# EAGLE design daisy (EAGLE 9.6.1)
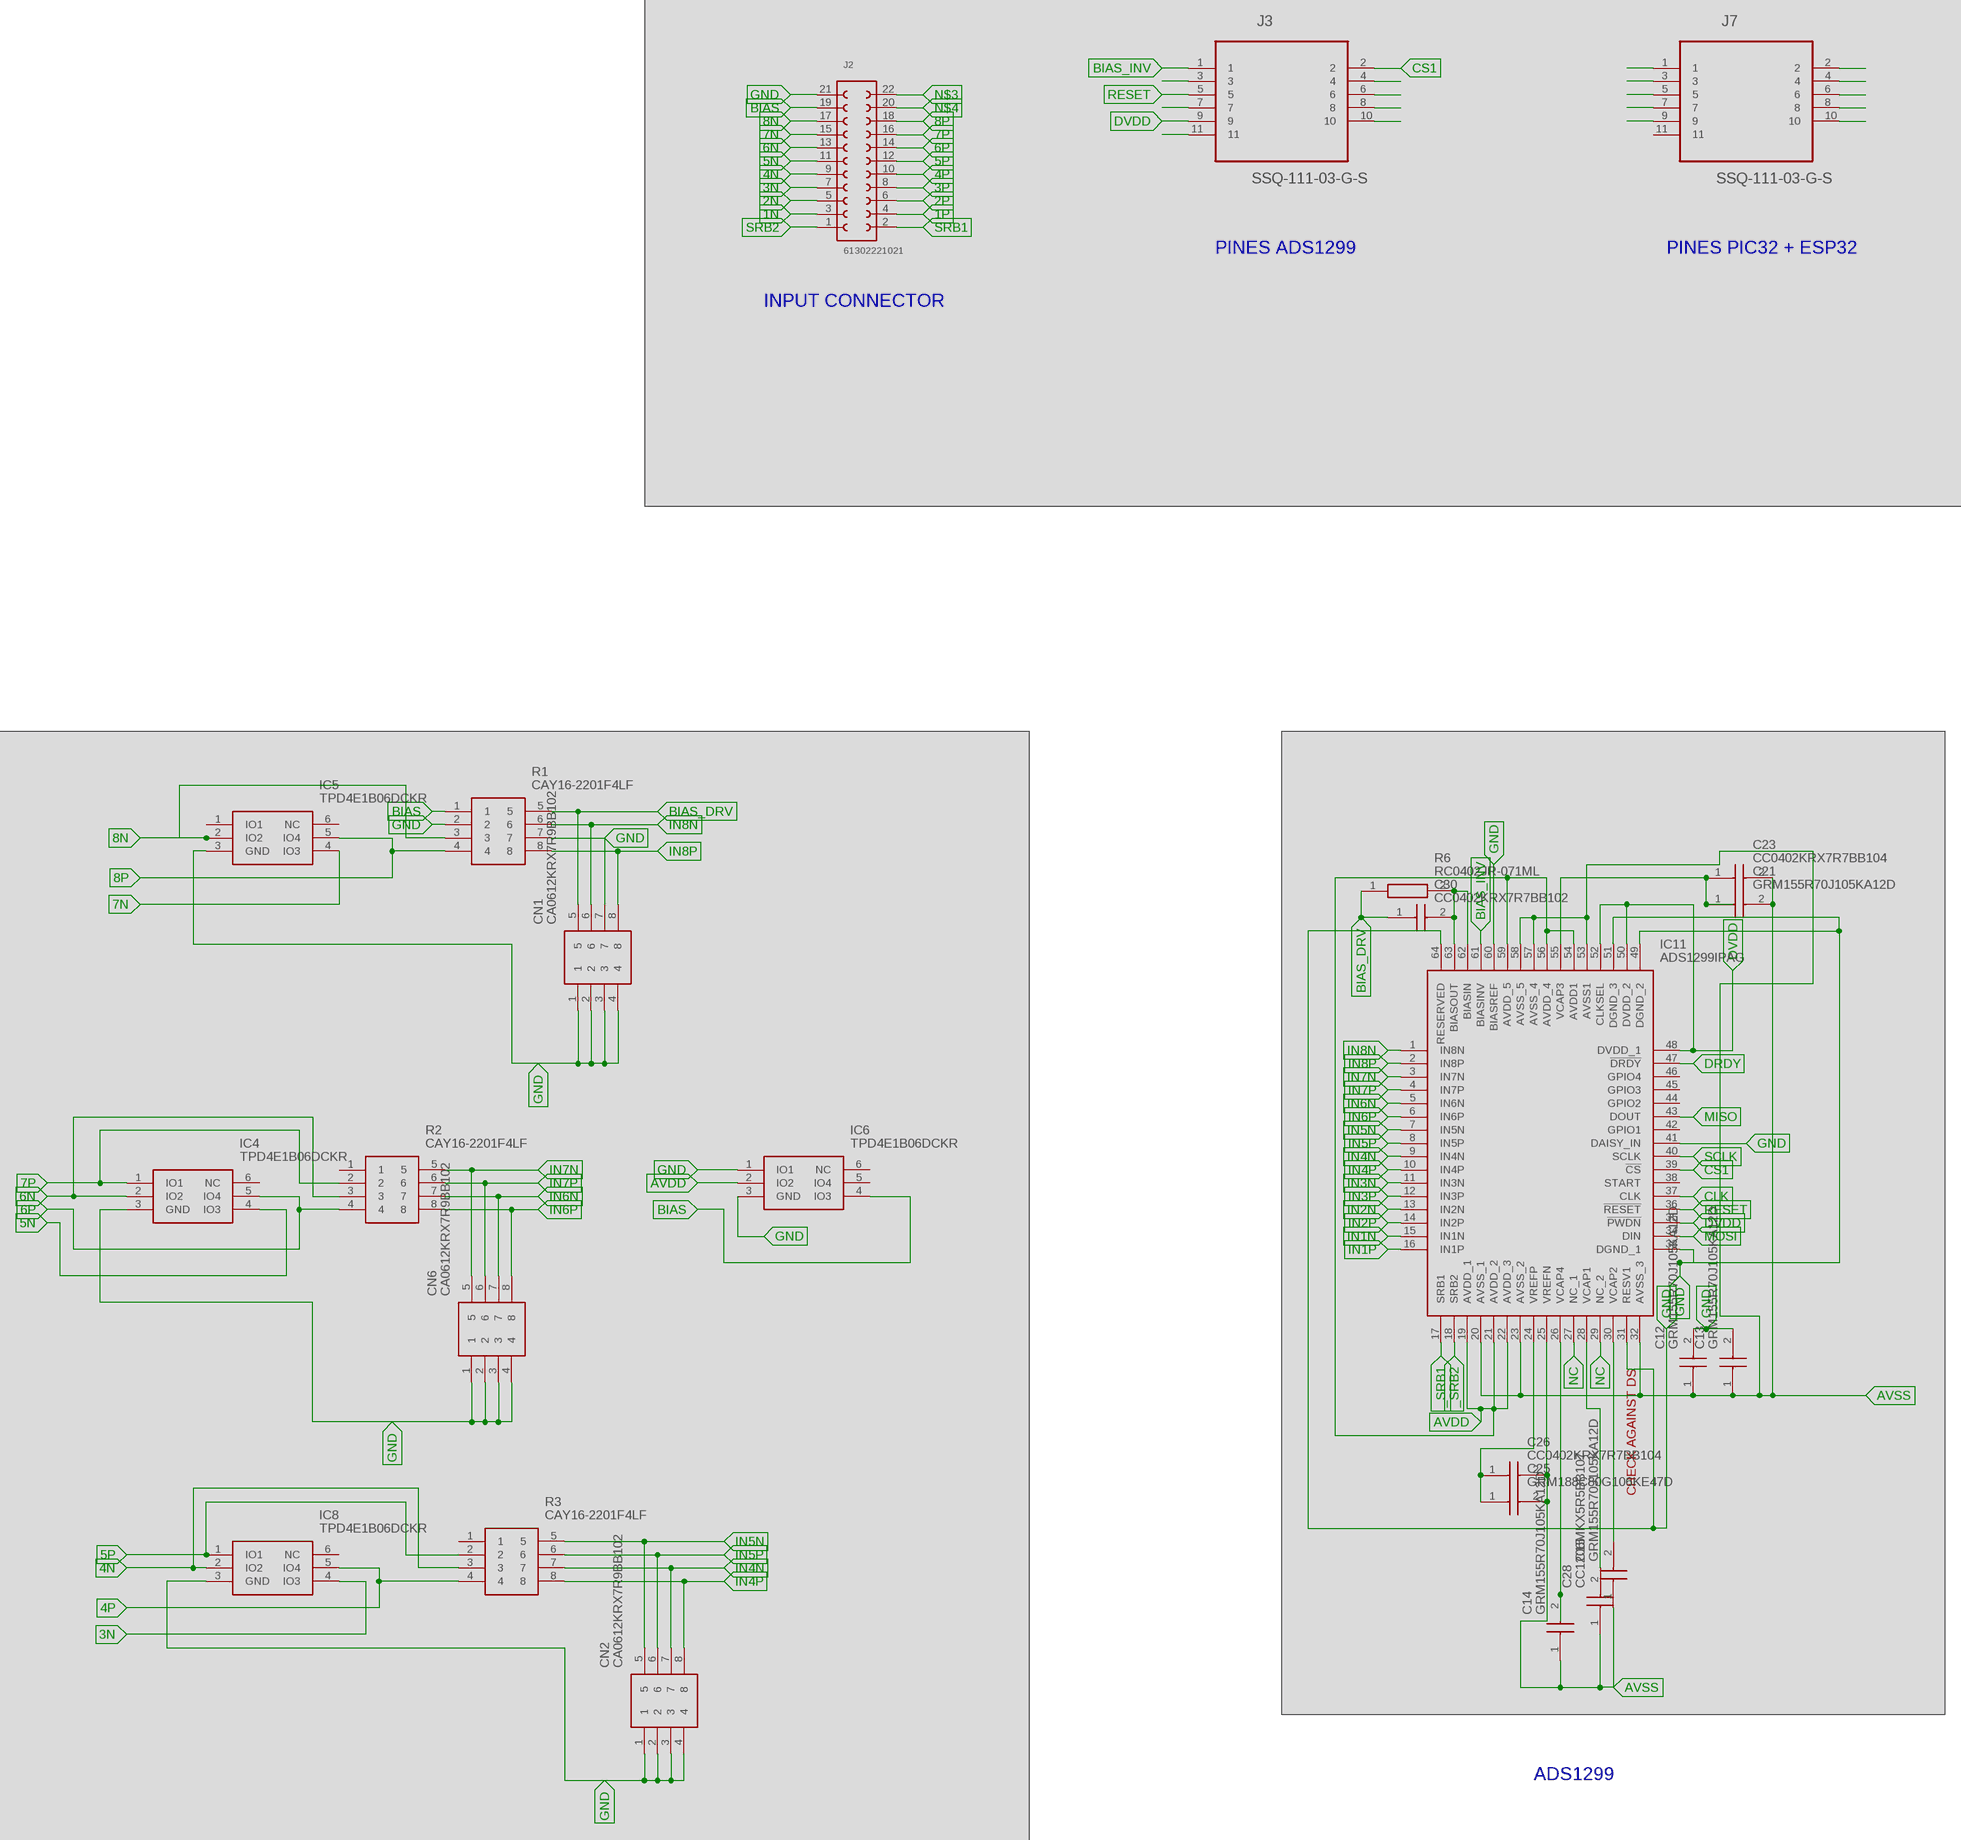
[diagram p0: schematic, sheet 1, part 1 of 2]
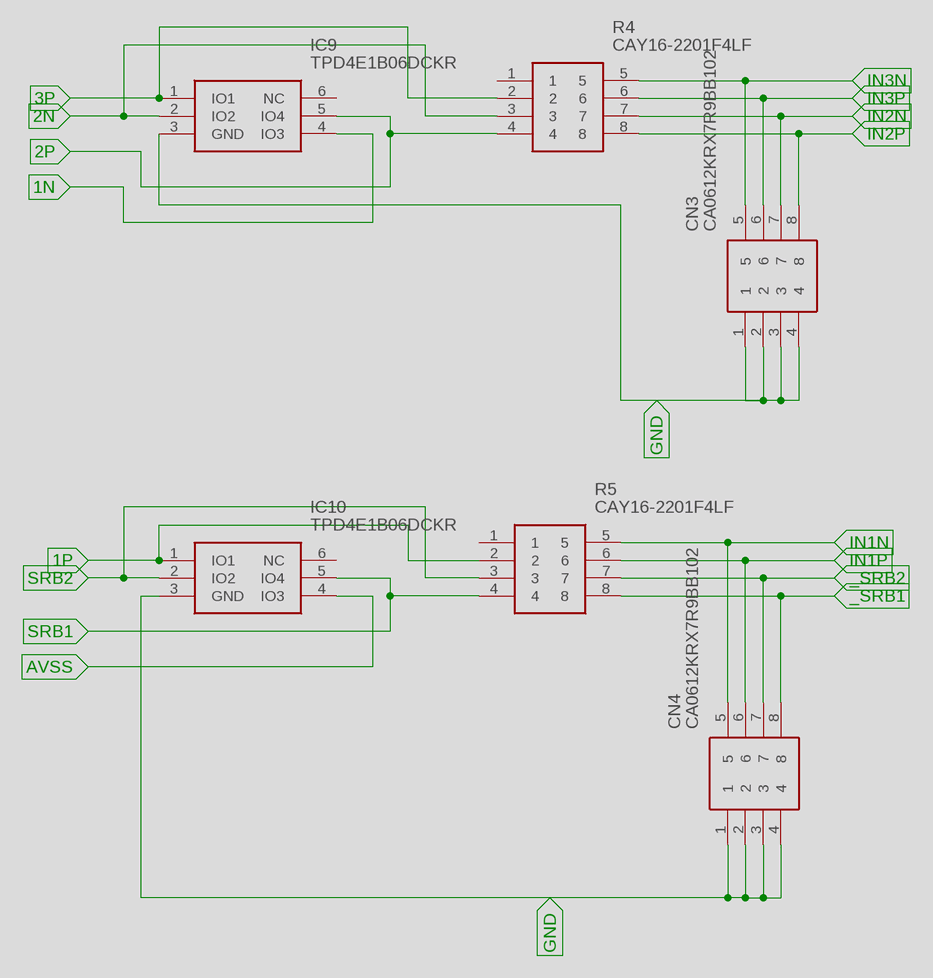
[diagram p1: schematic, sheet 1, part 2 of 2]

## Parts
C12  GRM155R70J105KA12D  [CAPC1005X55N]
C13  GRM155R70J105KA12D  [CAPC1005X55N]
C14  GRM155R70J105KA12D  [CAPC1005X55N]
C15  GRM155R70J105KA12D  [CAPC1005X55N]
C21  GRM155R70J105KA12D  [CAPC1005X55N]
C23  CC0402KRX7R7BB104  [CAPC1005X55N]
C25  GRM188C80G106KE47D  [CAPC1608X90N]
C26  CC0402KRX7R7BB104  [CAPC1005X55N]
C28  CC1206MKX5R5BB107  [CAPC3216X125N]
C30  CC0402KRX7R7BB102  [CAPC1005X55N]
CN1  CA0612KRX7R9BB102  [CA0612KRX7R9BB102]
CN2  CA0612KRX7R9BB102  [CA0612KRX7R9BB102]
CN3  CA0612KRX7R9BB102  [CA0612KRX7R9BB102]
CN4  CA0612KRX7R9BB102  [CA0612KRX7R9BB102]
CN6  CA0612KRX7R9BB102  [CA0612KRX7R9BB102]
IC4  TPD4E1B06DCKR  [SOT65P210X110-6N]
IC5  TPD4E1B06DCKR  [SOT65P210X110-6N]
IC6  TPD4E1B06DCKR  [SOT65P210X110-6N]
IC8  TPD4E1B06DCKR  [SOT65P210X110-6N]
IC9  TPD4E1B06DCKR  [SOT65P210X110-6N]
IC10  TPD4E1B06DCKR  [SOT65P210X110-6N]
IC11  ADS1299IPAG  [QFP50P1200X1200X120-64N]
J2  61302221021  [61302221021]
J3  SSQ-111-03-G-S  [SAMTEC_SSQ-111-03-G-S]
J7  SSQ-111-03-G-S  [SAMTEC_SSQ-111-03-G-S]
R1  CAY16-2201F4LF  [RESCAX80P160X320X60-8N]
R2  CAY16-2201F4LF  [RESCAX80P160X320X60-8N]
R3  CAY16-2201F4LF  [RESCAX80P160X320X60-8N]
R4  CAY16-2201F4LF  [RESCAX80P160X320X60-8N]
R5  CAY16-2201F4LF  [RESCAX80P160X320X60-8N]
R6  RC0402JR-071ML  [RESC1005X40N]

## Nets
1N: IC9.4(IO3) J2.3
1P: IC10.1(IO1) J2.4 R5.2
2N: IC9.2(IO2) J2.5 R4.3
2P: IC9.5(IO4) J2.6 R4.4
3N: IC8.4(IO3) J2.7
3P: IC9.1(IO1) J2.8 R4.2
3V3_ESP: J7.2
4N: IC8.2(IO2) J2.9 R3.3
4P: IC8.5(IO4) J2.10 R3.4
5N: IC4.4(IO3) J2.11
5P: IC8.1(IO1) J2.12 R3.2
6N: IC4.2(IO2) J2.13 R2.3
6P: IC4.5(IO4) J2.14 R2.4
7N: IC5.4(IO3) J2.15
7P: IC4.1(IO1) J2.16 R2.2
8N: IC5.2(IO2) J2.17 R1.3
8P: IC5.5(IO4) J2.18 R1.4
_SRB1: CN4.8 IC11.17(SRB1) R5.8
_SRB2: CN4.7 IC11.18(SRB2) R5.7
AVDD: IC6.2(IO2) IC11.19(AVDD_1) IC11.21(AVDD_2) IC11.22(AVDD_3) IC11.54(AVDD1) IC11.56(AVDD_4) IC11.59(AVDD_5) J3.10
AVSS: C12.1 C13.1 C14.1 C15.1 C21.2 C23.2 C25.2 C26.2 C28.1 IC10.4(IO3) IC11.20(AVSS_1) IC11.23(AVSS_2) IC11.25(VREFN) IC11.32(AVSS_3) IC11.53(AVSS1) IC11.57(AVSS_4) IC11.58(AVSS_5) J3.11
BIAS: IC6.4(IO3) J2.19 R1.1
BIAS_DRV: C30.1 CN1.5 R1.5 R6.1
BIAS_INV: IC11.61(BIASINV) J3.1
BOOT_EN: J3.6
CLK: IC11.37(CLK) J3.4
CS1: IC11.39(!CS) J3.2
CS2: J3.3
D13: J3.7
D18: J3.8
DRDY: IC11.47(!DRDY)
DVDD: IC11.35(!PWDN) IC11.48(DVDD_1) IC11.50(DVDD_2) IC11.52(CLKSEL) J3.9
GND: C12.2 C13.2 CN1.1 CN1.2 CN1.3 CN1.4 CN2.1 CN2.2 CN2.3 CN2.4 CN3.1 CN3.2 CN3.3 CN3.4 CN4.1 CN4.2 CN4.3 CN4.4 CN6.1 CN6.2 CN6.3 CN6.4 IC4.3(GND) IC5.3(GND) IC6.1(IO1) IC6.3(GND) IC8.3(GND) IC9.3(GND) IC10.3(GND) IC11.31(RESV1) IC11.33(DGND_1) IC11.41(DAISY_IN) IC11.49(DGND_2) IC11.51(DGND_3) IC11.60(BIASREF) IC11.64(RESERVED) J2.21 J7.3 R1.2
IN1N: CN4.5 IC11.15(IN1N) R5.5
IN1P: CN4.6 IC11.16(IN1P) R5.6
IN2N: CN3.7 IC11.13(IN2N) R4.7
IN2P: CN3.8 IC11.14(IN2P) R4.8
IN3N: CN3.5 IC11.11(IN3N) R4.5
IN3P: CN3.6 IC11.12(IN3P) R4.6
IN4N: CN2.7 IC11.9(IN4N) R3.7
IN4P: CN2.8 IC11.10(IN4P) R3.8
IN5N: CN2.5 IC11.7(IN5N) R3.5
IN5P: CN2.6 IC11.8(IN5P) R3.6
IN6N: CN6.7 IC11.5(IN6N) R2.7
IN6P: CN6.8 IC11.6(IN6P) R2.8
IN7N: CN6.5 IC11.3(IN7N) R2.5
IN7P: CN6.6 IC11.4(IN7P) R2.6
IN8N: CN1.6 IC11.1(IN8N) R1.6
IN8P: CN1.8 IC11.2(IN8P) R1.8
MCLR: J7.1
MISO: IC11.43(DOUT) J7.7
MOSI: IC11.34(DIN) J7.8
N$3: J2.22
N$4: J2.20
N$12: CN1.7 R1.7
N$36: C21.1 C23.1 IC11.55(VCAP3)
N$39: C25.1 C26.1 IC11.24(VREFP)
N$42: C28.2 IC11.28(VCAP1)
N$43: C15.2 IC11.30(VCAP2)
N$57: C30.2 IC11.62(BIASIN) IC11.63(BIASOUT) R6.2
N$97: C14.2 IC11.26(VCAP4)
NC: IC11.27(NC_1) IC11.29(NC_2)
PGC: J7.5
PGD: J7.4
RESET: IC11.36(!RESET) J3.5
RXD: J7.9
SCLK: IC11.40(SCLK) J7.6
SRB1: IC10.5(IO4) J2.2 R5.4
SRB2: IC10.2(IO2) J2.1 R5.3
TXD: J7.10
Unconnected: IC4.6(NC) IC5.1(IO1) IC5.6(NC) IC6.5(IO4) IC6.6(NC) IC8.6(NC) IC9.6(NC) IC10.6(NC) IC11.38(START) IC11.42(GPIO1) IC11.44(GPIO2) IC11.45(GPIO3) IC11.46(GPIO4) J7.11 R2.1 R3.1 R4.1 R5.1

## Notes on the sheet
- PINES ADS1299 | PINES PIC32 + ESP32
- INPUT CONNECTOR
- CHECK AGAINST DS
- ADS1299

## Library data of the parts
C12-C15 C21 = Cyton:GRM155R70J105KA12D: Multilayer Ceramic Capacitors MLCC - SMD/SMT 0402 1.0uF 6.3volts *Derate Voltage/Temp; DESCRIPTION: Multilayer Ceramic Capacitors MLCC - SMD/SMT 0402 1.0uF 6.3volts *Derate Voltage/Temp; HEIGHT: 0.55mm; MANUFACTURER_NAME: Murata Electronics; MANUFACTURER_PART_NUMBER: GRM155R70J105KA12D; RS_PART_NUMBER: 1138711P; RS_PRICE-STOCK: http://uk.rs-online.com/web/p/products/1138711P
C23 C26 = Cyton:CC0402KRX7R7BB104: Cap 100nF 16V 0402 SMD 10% X7R Phycomp 100nF Multilayer Ceramic Capacitor (MLCC) 16 V dc +/-10% X7R dielectric Standard max op. temp. +125C; DESCRIPTION: Cap 100nF 16V 0402 SMD 10% X7R Phycomp 100nF Multilayer Ceramic Capacitor (MLCC) 16 V dc +/-10% X7R dielectric Standard max op. temp. +125C; HEIGHT: 0.55mm; MANUFACTURER_NAME: YAGEO (PHYCOMP); MANUFACTURER_PART_NUMBER: CC0402KRX7R7BB104; RS_PART_NUMBER: 6169701; RS_PRICE-STOCK: https://uk.rs-online.com/web/p/products/6169701
C25 = Cyton:GRM188C80G106KE47D: Multilayer Ceramic Capacitors MLCC - SMD/SMT 0603 10uF 4volts *Derate Voltage/Temp; DESCRIPTION: Multilayer Ceramic Capacitors MLCC - SMD/SMT 0603 10uF 4volts *Derate Voltage/Temp; HEIGHT: 0.9mm; MANUFACTURER_NAME: Murata Electronics; MANUFACTURER_PART_NUMBER: GRM188C80G106KE47D; RS_PART_NUMBER: 1726485; RS_PRICE-STOCK: http://uk.rs-online.com/web/p/products/1726485
C28 = Cyton:CC1206MKX5R5BB107: Multilayer Ceramic Capacitors MLCC - SMD/SMT FACTORY NOT ACCEPTING ORDERS; DESCRIPTION: Multilayer Ceramic Capacitors MLCC - SMD/SMT FACTORY NOT ACCEPTING ORDERS; HEIGHT: 1.25mm; MANUFACTURER_NAME: YAGEO (PHYCOMP); MANUFACTURER_PART_NUMBER: CC1206MKX5R5BB107
C30 = Cyton:CC0402KRX7R7BB102: YAGEO - CC0402KRX7R7BB102 - CERAMIC CAPACITOR 1000PF, 16V, X7R, 10%, 0402, FULL REEL; DESCRIPTION: YAGEO - CC0402KRX7R7BB102 - CERAMIC CAPACITOR 1000PF, 16V, X7R, 10%, 0402, FULL REEL; HEIGHT: 0.55mm; MANUFACTURER_NAME: YAGEO (PHYCOMP); MANUFACTURER_PART_NUMBER: CC0402KRX7R7BB102
CN1-CN4 CN6 = Cyton:CA0612KRX7R9BB102: Capacitor,ceramic,multilayer,SMT,50V,1pF Source: Datasheet; DESCRIPTION: Capacitor,ceramic,multilayer,SMT,50V,1pF; HEIGHT: mm; MANUFACTURER_NAME: YAGEO (PHYCOMP); MANUFACTURER_PART_NUMBER: CA0612KRX7R9BB102; RS_PART_NUMBER: 6169789; RS_PRICE-STOCK: http://uk.rs-online.com/web/p/products/6169789
IC4-IC6 IC8-IC10 = Cyton:TPD4E1B06DCKR: Texas Instruments TPD4E1B06DCKR Quad Bi-Directional ESD Protection Array, 45W peak, 6-Pin SC-70 Source: Datasheet; DESCRIPTION: Texas Instruments TPD4E1B06DCKR Quad Bi-Directional ESD Protection Array, 45W peak, 6-Pin SC-70; HEIGHT: 1.1mm; MANUFACTURER_NAME: Texas Instruments; MANUFACTURER_PART_NUMBER: TPD4E1B06DCKR; RS_PART_NUMBER: 8255330P; RS_PRICE-STOCK: http://uk.rs-online.com/web/p/products/8255330P
IC11 = Cyton:ADS1299IPAG: Low-Noise, 8-Channel, 24-Bit Analog-to-Digital Converter for Biopotential Measurements Source: Datasheet; DESCRIPTION: Low-Noise, 8-Channel, 24-Bit Analog-to-Digital Converter for Biopotential Measurements; HEIGHT: 1.2mm; MANUFACTURER_NAME: Texas Instruments; MANUFACTURER_PART_NUMBER: ADS1299IPAG
J2 = Cyton:61302221021: WR-PHD 2.54mm Angled Dual Pin Header, 22 Pins =>Code : Con_BTB_PHD_2.54_2_61302221021 Details see: http://katalog.we-online.de/en/em/613_0xx_210_21 Created 2014-05-29, Karrer Zheng 2014 (C) Würth Elektronik; AVAILABILITY: Unavailable; DESCRIPTION: WR-PHD 2.54mm Angled Dual Pin Header 22p; MF: Wurth Electronics; MP: 61302221021; PACKAGE: None; PRICE: None
J3 J7 = Cyton:SSQ-111-03-G-S: CONN SOCKET, 2.54MM, THT VERT, 11POS; AVAILABILITY: Unavailable; DESCRIPTION: SSQ Series .100 Tiger Buy™ Socket Strip, Square Tail; MF: Samtec; MP: SSQ-111-03-G-S; PACKAGE: None; PRICE: None
R1-R5 = Cyton:CAY16-2201F4LF: Bourns CAY16 Series 2.2k +/-1% Isolated SMT Resistor Array, 4 Resistors, 0.25W total 1206 Package Convex Source: Datasheet; DESCRIPTION: Bourns CAY16 Series 2.2k +/-1% Isolated SMT Resistor Array, 4 Resistors, 0.25W total 1206 Package Convex; HEIGHT: 0.6mm; MANUFACTURER_NAME: Bourns; MANUFACTURER_PART_NUMBER: CAY16-2201F4LF; RS_PART_NUMBER: 7408773P; RS_PRICE-STOCK: http://uk.rs-online.com/web/p/products/7408773P
R6 = Cyton:RC0402JR-071ML: YAGEO RC0402 VALUE1; DESCRIPTION: YAGEO RC0402 VALUE1; HEIGHT: 0.4mm; MANUFACTURER_NAME: YAGEO (PHYCOMP); MANUFACTURER_PART_NUMBER: RC0402JR-071ML

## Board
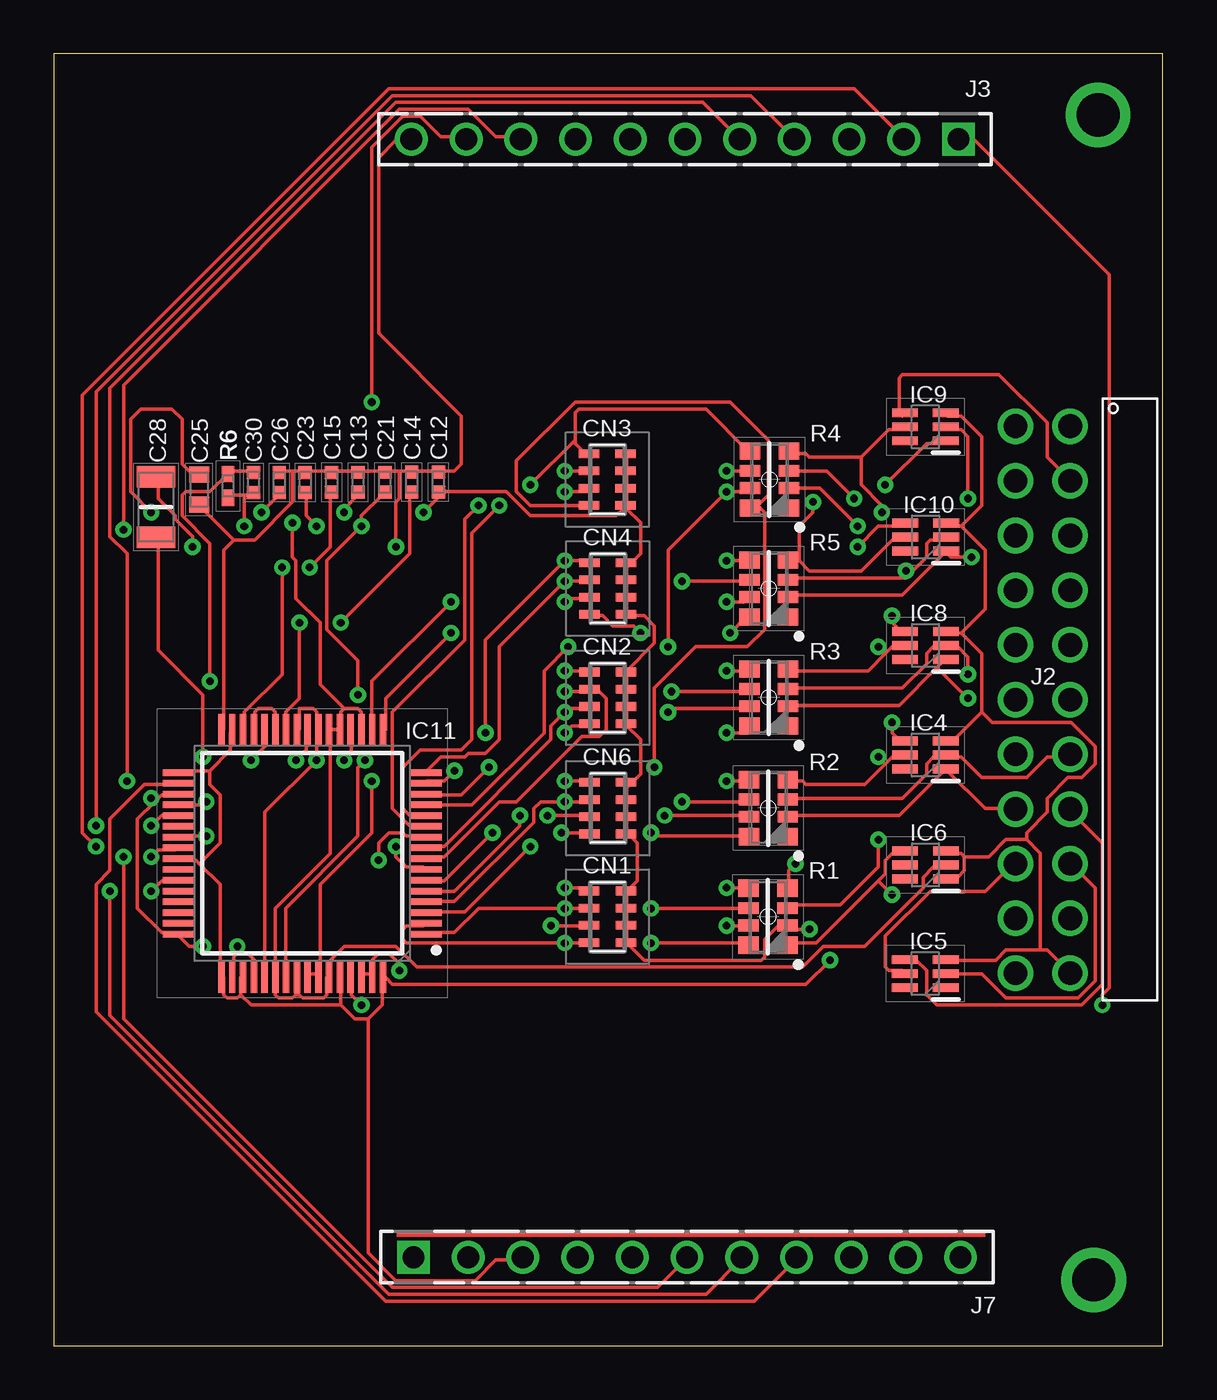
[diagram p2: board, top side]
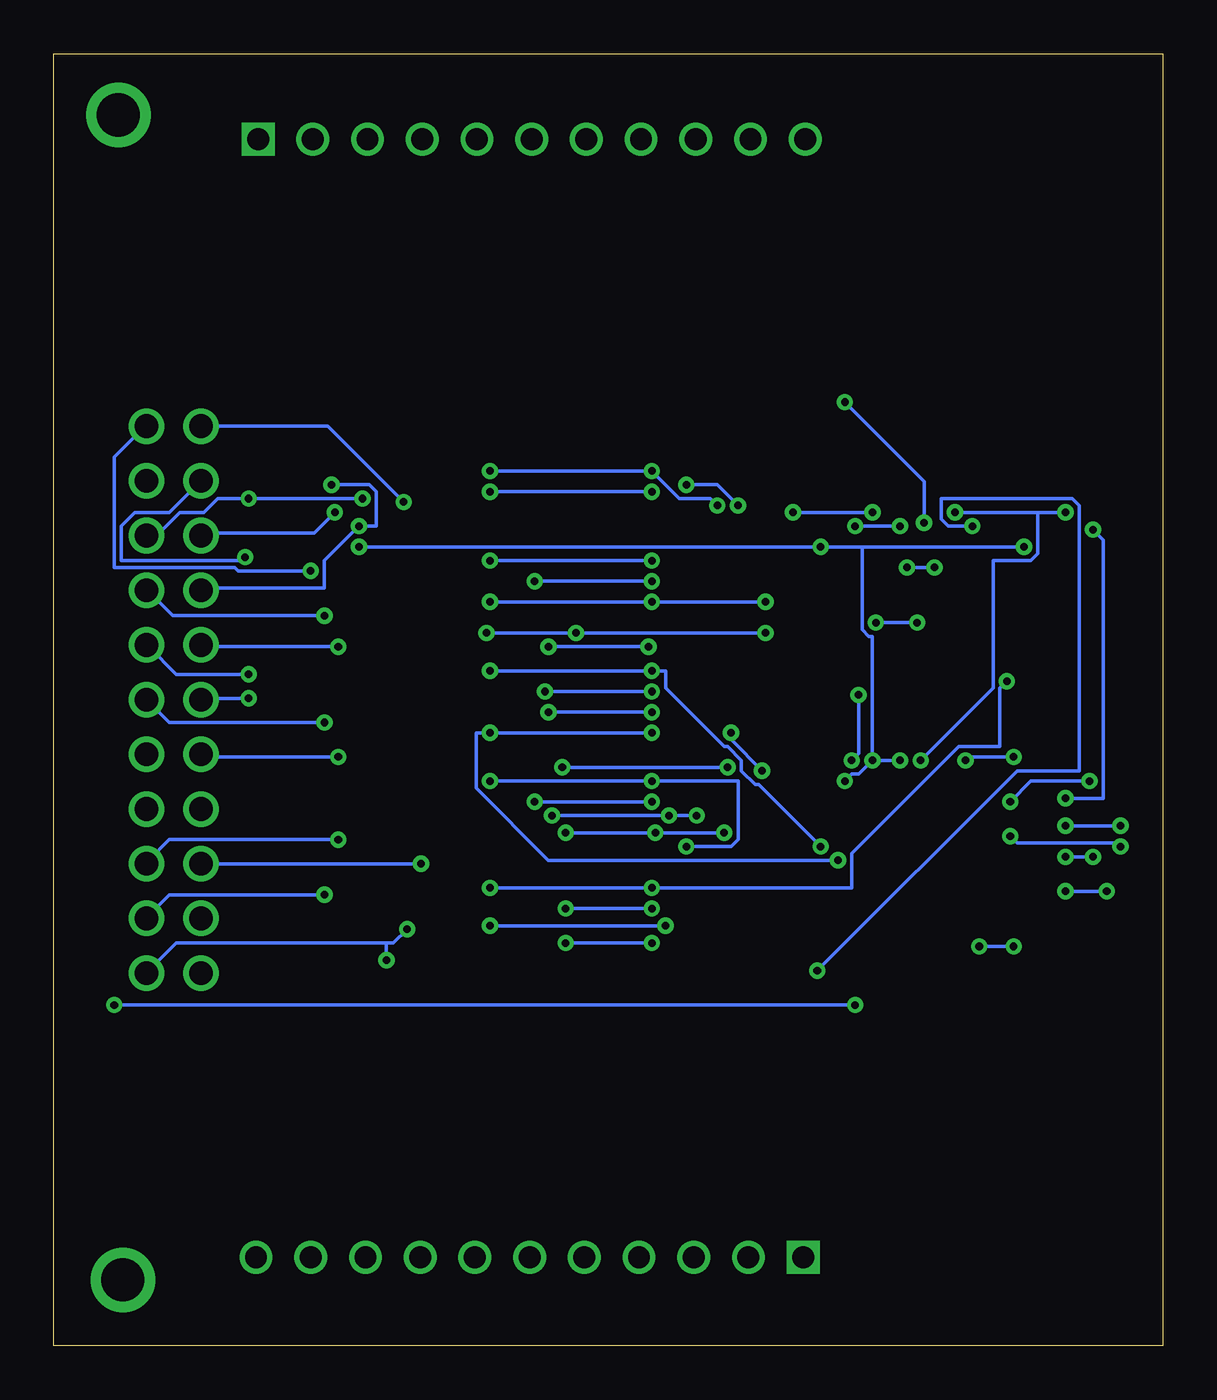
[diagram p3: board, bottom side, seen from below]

Size 51.48 x 60 mm. Coordinates in mm from the lower left corner, seen from the top.
Outline: 0,0 51.48,0 51.48,60 0,60 0,0
Copper layers (1*16): Top 0.035mm / dielectric 1.5mm / Bottom 0.035mm
Design rules "default *": minimum track width 6mil, minimum drill 0.35mm, track to track 6mil, track to pad 6mil, pad to pad 6mil, via to via 6mil, smd to smd 6mil, copper to edge 40mil, drill to drill 6mil, minimum pad ring 10mil, minimum via ring 8mil, stop-mask expansion 0mil, vias tented up to drill 100mil, thermal gap 10mil

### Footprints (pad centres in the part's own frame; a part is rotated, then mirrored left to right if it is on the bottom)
CAPC1005X55N = smd 0.6 x 0.62: 1 -0.46,0; 2 0.46,0
CAPC1608X90N = smd 0.75 x 0.94: 1 -0.7,0; 2 0.7,0
CAPC3216X125N = smd 0.99 x 1.78: 1 -1.4,0; 2 1.4,0
CA0612KRX7R9BB102 = smd 0.95 x 0.4: 1 -0.85,1.2; 2 -0.85,0.4; 3 -0.85,-0.4; 4 -0.85,-1.2; 5 0.85,-1.2; 6 0.85,-0.4; 7 0.85,0.4; 8 0.85,1.2
SOT65P210X110-6N = smd 1.2 x 0.4: 1 -0.95,0.65; 2 -0.95,0; 3 -0.95,-0.65; 4 0.95,-0.65; 5 0.95,0; 6 0.95,0.65
QFP50P1200X1200X120-64N = smd 1.475 x 0.3: 1 -5.738,3.75; 2 -5.738,3.25; 3 -5.738,2.75; 4 -5.738,2.25; 5 -5.738,1.75; 6 -5.738,1.25; 7 -5.738,0.75; 8 -5.738,0.25; 9 -5.738,-0.25; 10 -5.738,-0.75; 11 -5.738,-1.25; 12 -5.738,-1.75; 13 -5.738,-2.25; 14 -5.738,-2.75; 15 -5.738,-3.25; 16 -5.738,-3.75; 33 5.738,-3.75; 34 5.738,-3.25; 35 5.738,-2.75; 36 5.738,-2.25; 37 5.738,-1.75; 38 5.738,-1.25; 39 5.738,-0.75; 40 5.738,-0.25; 41 5.738,0.25; 42 5.738,0.75; 43 5.738,1.25; 44 5.738,1.75; 45 5.738,2.25; 46 5.738,2.75; 47 5.738,3.25; 48 5.738,3.75 | smd 0.3 x 1.475: 17 -3.75,-5.738; 18 -3.25,-5.738; 19 -2.75,-5.738; 20 -2.25,-5.738; 21 -1.75,-5.738; 22 -1.25,-5.738; 23 -0.75,-5.738; 24 -0.25,-5.738; 25 0.25,-5.738; 26 0.75,-5.738; 27 1.25,-5.738; 28 1.75,-5.738; 29 2.25,-5.738; 30 2.75,-5.738; 31 3.25,-5.738; 32 3.75,-5.738; 49 3.75,5.738; 50 3.25,5.738; 51 2.75,5.738; 52 2.25,5.738; 53 1.75,5.738; 54 1.25,5.738; 55 0.75,5.738; 56 0.25,5.738; 57 -0.25,5.738; 58 -0.75,5.738; 59 -1.25,5.738; 60 -1.75,5.738; 61 -2.25,5.738; 62 -2.75,5.738; 63 -3.25,5.738; 64 -3.75,5.738
61302221021 = drill 1.1: 1 12.7,-1.27; 2 12.7,1.27; 3 10.16,-1.27; 4 10.16,1.27; 5 7.62,-1.27; 6 7.62,1.27; 7 5.08,-1.27; 8 5.08,1.27; 9 2.54,-1.27; 10 2.54,1.27; 11 0,-1.27; 12 0,1.27; 13 -2.54,-1.27; 14 -2.54,1.27; 15 -5.08,-1.27; 16 -5.08,1.27; 17 -7.62,-1.27; 18 -7.62,1.27; 19 -10.16,-1.27; 20 -10.16,1.27; 21 -12.7,-1.27; 22 -12.7,1.27
SAMTEC_SSQ-111-03-G-S = drill 1.016 square: 1 -25.4,0 | drill 1.016: 2 -22.86,0; 3 -20.32,0; 4 -17.78,0; 5 -15.24,0; 6 -12.7,0; 7 -10.16,0; 8 -7.62,0; 9 -5.08,0; 10 -2.54,0; 11 0,0
RESCAX80P160X320X60-8N = smd 0.95 x 0.8: 1 -0.9,1.325; 4 -0.9,-1.325; 5 0.9,-1.325; 8 0.9,1.325 | smd 0.95 x 0.55: 2 -0.9,0.4; 3 -0.9,-0.4; 6 0.9,-0.4; 7 0.9,0.4
RESC1005X40N = smd 0.75 x 0.6: 1 -0.55,0; 2 0.55,0

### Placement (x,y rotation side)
C12  17.85,40.11 270 top
C13  14.12,40.1 270 top
C14  16.61,40.11 270 top
C15  12.9,40.1 270 top
C21  15.37,40.1 90 top
C23  11.67,40.09 90 top
C25  6.75,39.76 270 top
C26  10.47,40.08 90 top
C28  4.74,38.95 270 top
C30  9.27,40.09 270 top
CN1  25.71,19.92 180 top
CN2  25.71,30.09 180 top
CN3  25.7,40.22 180 top
CN4  25.72,35.16 180 top
CN6  25.72,24.96 180 top
IC4  40.46,27.43 180 top
IC5  40.46,17.29 180 top
IC6  40.47,22.33 180 top
IC8  40.47,32.52 180 top
IC9  40.46,42.67 180 top
IC10  40.48,37.56 180 top
IC11  11.53,22.87 180 top
J2  45.92,30.01 90 top
J3  16.6,56.04 180 top
J7  42.1,4.11 0 top
R1  33.16,19.92 180 top
R2  33.17,24.96 180 top
R3  33.19,30.1 180 top
R4  33.23,40.23 180 top
R5  33.19,35.17 180 top
R6  8.09,39.93 270 top

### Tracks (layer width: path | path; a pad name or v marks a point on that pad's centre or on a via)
1N
  Top 0.152: IC9.4 39.4,43.18 39.24,43.34 39.24,44.94 39.4,45.1 43.88,45.1 46.12,42.86 46.12,41.26 47.08,40.3 J2.3
1P  (via drill 0.35)
  Top 0.152: R5.2 34.12,34.86 39.4,34.86 41.32,36.78 IC10.1 41.48,36.78 41.64,36.62 v42.6,36.62
  Bottom 0.152: v42.6,36.62 42.76,36.46 48.36,36.46 48.36,38.06 47.72,38.7 46.12,38.7 44.68,40.14 J2.4
2N  (via drill 0.35)
  Top 0.152: v37.16,39.34 35.88,40.62 34.28,40.62 R4.3 | v42.44,39.34 42.44,42.22 42.12,42.54 41.48,42.54 IC9.2
  Bottom 0.152: v37.16,39.34 v42.44,39.34 43.88,39.34 44.52,38.7 45.64,38.7 46.6,37.74 47.08,37.74 J2.5
2P  (via drill 0.35)
  Top 0.152: 37.48,41.26 35.08,41.26 34.92,41.42 34.28,41.42 R4.4 | 37.48,41.26 38.76,42.54 39.4,42.54 IC9.5 | 37.48,41.26 37.48,39.98 38.44,39.02 v38.44,38.7
  Bottom 0.152: v38.44,38.7 39.4,37.74 44.52,37.74 J2.6
3N  (via drill 0.35)
  Top 0.152: v38.92,33.9 38.92,33.58 39.4,33.1 IC8.4
  Bottom 0.152: v38.92,33.9 45.96,33.9 47.08,35.02 J2.7
3P  (via drill 0.35)
  Top 0.152: v37.32,38.06 35.56,39.82 34.28,39.82 R4.2 | v38.6,39.98 40.52,41.9 41.32,41.9 IC9.1
  Bottom 0.152: J2.8 44.52,35.18 38.92,35.18 38.92,36.46 v37.32,38.06 36.52,38.06 36.52,39.66 36.84,39.98 v38.6,39.98
4N  (via drill 0.35)
  Top 0.152: R3.3 34.12,30.54 39.4,30.54 40.52,31.66 40.52,32.14 40.84,32.46 41.32,32.46 IC8.2 41.48,32.46 41.96,32.46 42.44,31.98 v42.44,31.18
  Bottom 0.152: v42.44,31.18 45.8,31.18 47.08,32.46 J2.9
4P  (via drill 0.35)
  Top 0.152: 38.6,32.14 38.92,32.46 39.4,32.46 IC8.5 | 38.6,32.14 37.8,31.34 34.12,31.34 R3.4 | v38.28,32.46 38.6,32.14
  Bottom 0.152: v38.28,32.46 44.52,32.46 J2.10
5N  (via drill 0.35)
  Top 0.152: v38.92,28.94 38.92,28.46 39.4,27.98 IC4.4
  Bottom 0.152: v38.92,28.94 46.12,28.94 47.08,29.9 J2.11
5P  (via drill 0.35)
  Top 0.152: 41,31.5 41.32,31.82 IC8.1 | 41,31.5 39.24,29.74 34.12,29.74 R3.2 | 41,31.5 v42.44,30.06
  Bottom 0.152: v42.44,30.06 44.52,30.06 J2.12
6N
  Top 0.152: R2.3 34.12,25.42 39.4,25.42 40.52,26.54 40.52,27.02 40.84,27.34 41.32,27.34 IC4.2 41.48,27.34 42.12,27.34 43.08,26.38 45.16,26.38 46.12,27.34 47.08,27.34 J2.13
6P  (via drill 0.35)
  Top 0.152: 38.6,27.02 38.92,27.34 39.4,27.34 IC4.5 | 38.6,27.02 37.64,26.06 34.92,26.06 34.76,26.22 34.12,26.22 R2.4 | v38.28,27.34 38.6,27.02
  Bottom 0.152: v38.28,27.34 44.52,27.34 J2.14
7N
  Top 0.152: IC5.4 39.56,17.9 40.04,17.9 40.52,17.42 40.52,16.3 41,15.82 47.72,15.82 48.68,16.78 48.68,23.34 47.24,24.78 J2.15
7P
  Top 0.152: R2.2 34.12,24.62 39.24,24.62 41.32,26.7 IC4.1 41.48,26.7 43.24,24.94 44.52,24.94 J2.16
8N  (via drill 0.35)
  Top 0.152: v38.28,23.5 38.28,22.22 36.52,20.46 34.12,20.46 R1.3 | IC5.2 41.48,17.26 43.08,17.26 44.2,16.14 47.56,16.14 48.36,16.94 48.36,21.26 47.24,22.38 J2.17
  Bottom 0.152: v38.28,23.5 46.12,23.5 47.08,22.54 J2.17
8P  (via drill 0.35)
  Top 0.152: v34.44,22.38 34.12,22.06 34.12,21.26 R1.4 | IC5.5 39.4,17.42 38.76,17.42 38.6,17.58 38.6,19.02 40.68,21.1 43.24,21.1 44.52,22.38 J2.18
  Bottom 0.152: v34.44,22.38 44.52,22.38 J2.18
_SRB1  (via drill 0.35)
  Top 0.152: v27.24,33.1 26.92,33.42 25.96,33.42 25.48,33.9 25,33.9 CN4.8 | v31.4,33.1 32.2,33.9 R5.8 | v18.44,33.1 15.4,30.06 15.4,28.62 IC11.17
  Bottom 0.152: v31.4,33.1 v27.24,33.1 v18.44,33.1
_SRB2  (via drill 0.35)
  Top 0.152: v23.72,34.54 23.88,34.7 24.84,34.7 CN4.7 | v31.24,34.54 32.04,34.54 32.2,34.7 R5.7 | v18.44,34.54 14.76,30.86 14.76,28.62 IC11.18
  Bottom 0.152: v31.24,34.54 v23.72,34.54 v18.44,34.54
AVDD  (via drill 0.35)
  Top 0.152: 13.48,29.58 14.12,29.58 14.28,29.42 14.28,28.62 IC11.19 | 13.48,29.58 13.32,29.42 13.32,28.62 IC11.21 13.16,28.62 12.84,28.62 IC11.22 12.84,28.46 12.84,22.86 10.28,20.3 10.28,17.26 IC11.54 10.28,17.1 10.28,16.3 10.44,16.14 11.08,16.14 11.24,16.3 | 11.24,16.3 11.24,17.1 IC11.56 | IC6.2 41.32,22.22 40.84,22.22 40.36,21.74 40.36,21.26 37.64,18.54 35.72,18.54 34.76,17.58 16.84,17.58 15.88,18.54 13.48,18.54 12.84,17.9 12.84,17.26 IC11.59 12.68,17.1 12.68,16.3 12.52,16.14 11.56,16.14 11.4,16.3 11.24,16.3 | v14.76,43.82 14.76,55.66 16.2,57.1 17,57.1 17.96,56.14 19.08,56.14 J3.10 | v11.08,38.22 11.08,36.62 11.24,36.46 11.24,34.7 12.36,33.58 12.36,30.7 13.48,29.58
  Bottom 0.152: v14.76,43.82 11.08,40.14 v11.08,38.22
AVSS  (via drill 0.35)
  Top 0.152: IC11.57 11.88,17.26 12.2,17.26 IC11.58 12.36,17.26 12.36,21.42 14.76,23.82 v14.76,26.22 | IC11.53 9.8,17.26 9.8,24.78 v12.2,27.18 12.2,28.46 IC11.23 12.2,28.62 12.2,29.42 12.04,29.58 11.4,29.58 11.4,28.62 IC11.25 | v13.48,27.18 13.8,27.5 13.8,28.46 IC11.20 | 11.08,40.62 11.56,40.62 C23.2 11.72,40.62 12.84,40.62 C15.1 13,40.62 14.12,40.62 C13.1 14.28,40.62 15.24,40.62 C21.2 15.4,40.62 16.04,40.62 | 11.08,40.62 10.6,40.62 C26.2 | 8.36,37.42 6.76,39.02 C25.2 | 8.36,37.42 9.32,37.42 11.08,39.18 11.08,40.62 | 8.36,37.42 7.88,36.94 7.88,28.62 IC11.32 | 16.04,40.62 16.52,40.62 C14.1 16.68,40.62 17.8,40.62 C12.1 17.96,40.62 18.6,40.62 18.92,40.94 18.92,43.18 15.08,47.02 15.08,55.18 15.88,55.98 16.52,55.98 J3.11 | v37.32,37.1 38.28,38.06 39.4,38.06 IC10.4 | v15.88,37.1 15.88,39.18 16.04,39.34 16.04,40.62 | v6.44,37.1 6.44,37.58 5.64,38.38 5.64,38.54 4.84,39.34 4.84,40.3 C28.1
  Bottom 0.152: v12.2,27.18 v13.48,27.18 | v14.76,26.22 14.44,26.54 14.12,26.54 v13.48,27.18 | v37.32,37.1 v15.88,37.1 13.96,37.1 | 13.96,37.1 v6.44,37.1 | v13.48,27.18 13.48,32.94 13.64,32.94 13.96,33.26 13.96,37.1
BIAS  (via drill 0.35)
  Top 0.152: 38.28,21.58 38.6,21.9 38.6,22.54 38.92,22.86 39.4,22.86 IC6.4 | 38.28,21.58 35.4,18.7 34.12,18.7 R1.1 | 38.28,21.58 v38.92,20.94
  Bottom 0.152: v38.92,20.94 46.12,20.94 47.08,19.98 J2.19
BIAS_DRV  (via drill 0.35)
  Top 0.152: C30.1 9.16,40.62 8.2,40.62 R6.1 8.04,40.46 7.24,39.66 6.12,39.66 5.96,39.5 5.96,38.54 7.24,37.26 v7.24,30.86 | v23.72,21.26 24.84,21.26 CN1.5 | v31.24,21.26 32.2,21.26 R1.5
  Bottom 0.152: v31.24,21.26 v23.72,21.26 14.44,21.26 14.44,22.86 9.48,27.82 7.56,27.82 7.56,30.54 v7.24,30.86
BIAS_INV  (via drill 0.35)
  Top 0.152: v14.28,15.82 13.8,16.3 13.8,17.1 IC11.61 | v48.68,15.82 48.68,16.3 49,16.62 49,49.74 42.76,55.98 42.12,55.98 J3.1
  Bottom 0.152: v48.68,15.82 v14.28,15.82
CLK  (via drill 0.35)
  Top 0.152: v4.52,24.14 5,24.62 5.64,24.62 IC11.37 | v1.96,24.14 1.96,44.3 15.72,58.06 32.36,58.06 34.28,56.14 J3.4
  Bottom 0.152: v1.96,24.14 v4.52,24.14
CS1  (via drill 0.35)
  Top 0.152: v7.08,23.66 5.8,23.66 IC11.39 | v1.96,23.18 1.32,23.82 1.32,44.14 15.56,58.38 37.16,58.38 39.4,56.14 J3.2
  Bottom 0.152: v7.08,23.66 6.76,23.34 2.12,23.34 v1.96,23.18
DVDD  (via drill 0.35)
  Top 0.152: 8.52,18.22 8.36,18.06 8.36,17.26 IC11.50 | 8.52,18.22 9,18.22 9.32,17.9 9.32,17.26 IC11.52 | 4.68,25.26 5,25.58 5.64,25.58 IC11.35 | 4.68,25.26 3.88,24.46 3.88,20.3 5,19.18 5.64,19.18 IC11.48 5.8,19.02 6.28,18.54 v6.92,18.54 | v8.52,18.54 8.52,18.22 | v3.24,37.9 3.24,44.62 16.04,57.42 19.24,57.42 20.52,56.14 21.64,56.14 J3.9 | 4.68,25.26 v4.52,25.42
  Bottom 0.152: v6.92,18.54 v8.52,18.54 | v3.24,37.9 2.76,37.42 2.76,25.42 v4.52,25.42
GND  (via drill 0.35)
  Top 0.152: 7.24,26.7 5.8,26.7 IC11.33 | 7.24,26.7 8.2,27.66 8.2,28.46 IC11.31 | 13.32,15.82 13.32,17.1 IC11.60 | 13.32,15.82 13.96,15.18 14.6,15.18 | 14.6,15.18 15.24,15.82 15.24,17.1 IC11.64 15.4,17.1 15.72,16.78 34.92,16.78 v36.04,17.9 | 8.68,16.3 8.52,16.14 8.04,16.14 7.88,16.3 7.88,17.1 IC11.49 7.72,17.26 7.72,21.42 6.76,22.38 | 8.68,16.3 8.68,17.1 IC11.51 | 6.76,22.38 6.6,22.54 5.8,22.54 IC11.41 | 13.32,15.82 9.16,15.82 8.68,16.3 | 7.24,26.7 7.24,26.06 7.72,25.58 7.72,23.34 6.76,22.38 | 14.6,15.18 14.6,4.3 15.88,3.02 19.56,3.02 20.52,3.98 21.64,3.98 J7.3 | 42.28,22.7 42.28,22.06 41.96,21.74 41.48,21.74 IC6.1 | 42.28,22.7 42.12,22.86 41.48,22.86 IC6.3 | 45.8,18.38 46.12,18.38 47.08,17.42 J2.21 | 45.8,18.38 44.2,18.38 43.72,17.9 41.48,17.9 IC5.3 | 42.28,22.7 43.4,22.7 44.2,23.5 45.16,23.5 | 45.16,23.5 45.8,22.86 45.8,18.38 | 43.08,29.42 41.64,27.98 41.48,27.98 IC4.3 | 43.08,29.42 43.08,32.14 42.12,33.1 | 42.12,33.1 41.48,33.1 IC8.3 | 42.12,38.06 41.48,38.06 IC10.3 | 42.12,38.06 43.24,36.94 43.24,34.22 42.12,33.1 | 42.12,38.06 43.08,39.02 43.08,42.22 42.12,43.18 41.48,43.18 IC9.3 | 45.16,23.5 45.16,23.82 46.12,24.78 46.12,25.42 47.08,26.38 47.72,26.38 48.36,27.02 48.36,27.82 47.24,28.94 43.56,28.94 43.08,29.42 | 26.6,25.9 26.6,26.06 CN6.4 | 26.6,25.9 26.6,25.42 CN6.3 26.6,25.26 26.6,24.62 CN6.2 26.6,24.46 26.6,23.82 CN6.1 26.6,23.66 26.76,23.66 27.08,23.34 27.08,21.58 26.6,21.1 | 26.6,21.1 26.6,20.46 CN1.3 26.6,20.3 26.6,19.66 CN1.2 26.6,19.5 26.6,18.86 CN1.1 26.6,18.7 27.4,17.9 32.84,17.9 33,18.06 33,18.86 33.64,19.5 33.96,19.5 R1.2 34.12,19.5 34.28,19.34 v35.08,19.34
  Top 0.152: 26.6,21.1 CN1.4 | 26.6,25.9 27.24,26.54 27.24,28.14 26.6,28.78 CN2.1 26.6,28.94 26.6,29.58 CN2.2 26.6,29.74 26.6,30.38 CN2.3 26.6,30.54 26.6,31.18 CN2.4 26.6,31.34 27.88,32.62 27.88,33.42 27.4,33.9 26.6,33.9 CN4.1 26.6,34.06 26.6,34.7 CN4.2 26.6,34.86 26.6,35.5 CN4.3 26.6,35.66 26.6,36.14 | v13.48,38.7 13.48,38.86 14.12,39.5 C13.2 | v17.16,38.7 17.96,39.5 C12.2 17.96,39.66 21,39.66 22.12,38.54 26.12,38.54 26.44,38.86 CN3.1 | CN3.1 26.6,39.02 26.6,39.66 CN3.2 26.6,39.82 26.6,40.46 CN3.3 26.6,40.62 26.6,41.26 CN3.4 | 26.6,36.14 26.6,36.3 CN4.4 | 26.6,36.14 27.24,36.78 27.24,38.22 26.6,38.86 CN3.1
  Bottom 0.152: v17.16,38.7 v13.48,38.7 | 36.04,18.7 35.72,18.7 v35.08,19.34 | 36.04,18.7 45.8,18.7 47.08,17.42 J2.21 | 36.04,18.7 v36.04,17.9
IN1N  (via drill 0.35)
  Top 0.152: v31.24,36.46 32.2,36.46 R5.5 | CN4.5 24.84,36.46 v23.72,36.46 20.04,32.78 v20.04,28.46 | v18.6,26.7 18.12,26.22 17.32,26.22 IC11.15
  Bottom 0.152: v31.24,36.46 v23.72,36.46 | v18.6,26.7 20.04,28.14 v20.04,28.46
IN1P  (via drill 0.35)
  Top 0.152: CN4.6 24.84,35.5 v23.72,35.5 20.68,32.46 20.68,28.14 20.04,27.5 19.24,27.5 19.08,27.34 17.96,27.34 17.32,26.7 IC11.16 | v29.16,35.5 32.2,35.5 R5.6
  Bottom 0.152: v23.72,35.5 v29.16,35.5
IN2N  (via drill 0.35)
  Top 0.152: v23.72,39.66 24.84,39.66 CN3.7 | R4.7 32.2,39.82 32.04,39.66 v31.24,39.66 28.52,36.94 v28.52,32.46 | v23.88,32.46 22.76,31.34 22.76,28.46 19.4,25.1 17.32,25.1 IC11.13
  Bottom 0.152: v31.24,39.66 v23.72,39.66 | v28.52,32.46 v23.88,32.46
IN2P  (via drill 0.35)
  Top 0.152: 32.68,39.02 32.36,39.02 R4.8 32.68,39.02 | 32.68,39.02 33.16,39.5 33.16,42.06 31.4,43.82 24.2,43.82 21.48,41.1 21.48,39.66 22.12,39.02 CN3.8 | v20.2,26.86 18.92,25.58 17.32,25.58 IC11.14 | v27.88,26.86 27.88,30.54 29.8,32.46 32.2,32.46 33,33.26 33,38.7 32.68,39.02
  Bottom 0.152: v27.88,26.86 v20.2,26.86
IN3N  (via drill 0.35)
  Top 0.152: 24.2,42.06 24.2,43.34 24.36,43.5 30.28,43.5 32.2,41.58 R4.5 | 24.2,42.06 24.2,41.9 24.68,41.42 CN3.5 | v19.72,39.02 19.08,38.38 19.08,32.78 15.72,29.42 15.72,24.94 16.52,24.14 17.16,24.14 IC11.11 | 24.2,42.06 v22.12,39.98
  Bottom 0.152: v19.72,39.02 20.68,39.98 v22.12,39.98
IN3P  (via drill 0.35)
  Top 0.152: v23.72,40.62 CN3.6 | v31.24,40.62 32.2,40.62 R4.6 | v20.68,39.02 19.4,37.74 19.4,28.14 18.92,27.66 17,27.66 16.2,26.86 16.2,24.94 16.52,24.62 17.16,24.62 IC11.12
  Bottom 0.152: v31.24,40.62 v23.72,40.62 22.44,39.34 21,39.34 v20.68,39.02
IN4N  (via drill 0.35)
  Top 0.152: CN2.7 24.84,29.58 23.88,29.58 v23.72,29.42 23.08,28.78 23.08,28.14 18.12,23.18 17.32,23.18 IC11.9 | v28.52,29.42 28.68,29.58 32.2,29.58 R3.7
  Bottom 0.152: v23.72,29.42 v28.52,29.42
IN4P  (via drill 0.35)
  Top 0.152: v23.72,28.46 24.04,28.78 24.84,28.78 CN2.8 | v31.24,28.46 32.04,28.46 32.2,28.62 R3.8 | v15.08,22.54 15.08,23.34 15.56,23.82 16.2,23.82 16.36,23.66 17.16,23.66 IC11.10
  Bottom 0.152: v23.72,28.46 v31.24,28.46 31.88,28.46 31.88,25.9 28.52,22.54 v15.08,22.54
IN5N  (via drill 0.35)
  Top 0.152: v23.72,31.34 24.84,31.34 CN2.5 | v31.24,31.34 32.2,31.34 R3.5 | v15.88,23.18 15.88,22.7 16.36,22.22 17.16,22.22 IC11.7
  Bottom 0.152: v31.24,31.34 v23.72,31.34 23.08,31.34 23.08,30.54 20.36,27.82 20.2,27.82 19.56,27.18 19.56,26.7 18.92,26.06 18.76,26.06 v15.88,23.18
IN5P  (via drill 0.35)
  Top 0.152: IC11.8 17.32,22.7 18.12,22.7 20.68,25.26 21.48,25.26 24.52,28.3 25.32,28.3 25.64,28.62 25.64,30.06 25.32,30.38 25,30.38 CN2.6 24.84,30.38 v23.72,30.38 | v28.68,30.38 32.2,30.38 R3.6
  Bottom 0.152: v23.72,30.38 v28.68,30.38
IN6N  (via drill 0.35)
  Top 0.152: v22.92,24.62 24.84,24.62 CN6.7 | v21.64,24.62 21.64,24.14 18.6,21.1 17.32,21.1 IC11.5 | v28.36,24.62 32.2,24.62 R2.7
  Bottom 0.152: v21.64,24.62 v22.92,24.62 v28.36,24.62
IN6P  (via drill 0.35)
  Top 0.152: v23.56,23.82 24.84,23.82 CN6.8 | v20.36,23.82 18.12,21.58 17.32,21.58 IC11.6 | v27.72,23.82 27.88,23.66 32.2,23.66 R2.8
  Bottom 0.152: v20.36,23.82 v23.56,23.82 v27.72,23.82
IN7N  (via drill 0.35)
  Top 0.152: v23.72,26.22 24.84,26.22 CN6.5 | v31.24,26.22 32.2,26.22 R2.5 | v22.12,23.18 19.08,20.14 17.32,20.14 IC11.3
  Bottom 0.152: v31.24,26.22 v23.72,26.22 19.72,26.22 19.72,23.5 20.04,23.18 v22.12,23.18
IN7P  (via drill 0.35)
  Top 0.152: CN6.6 24.84,25.26 v23.72,25.26 22.6,25.26 22.28,24.94 22.28,24.3 18.6,20.62 17.32,20.62 IC11.4 | v29.16,25.26 32.2,25.26 R2.6
  Bottom 0.152: v23.72,25.26 v29.16,25.26
IN8N  (via drill 0.35)
  Top 0.152: CN1.6 24.84,20.3 v23.72,20.3 19.72,20.3 18.6,19.18 17.32,19.18 IC11.1 | v27.72,20.3 32.2,20.3 R1.6
  Bottom 0.152: v23.72,20.3 v27.72,20.3
IN8P  (via drill 0.35)
  Top 0.152: CN1.8 24.84,18.7 v23.72,18.7 16.36,18.7 16.2,18.86 16.2,19.34 16.36,19.5 17.16,19.5 IC11.2 | v27.72,18.7 32.2,18.7 R1.8
  Bottom 0.152: v23.72,18.7 v27.72,18.7
MISO  (via drill 0.35)
  Top 0.152: v4.52,21.1 5,21.58 5.64,21.58 IC11.43 | v2.6,21.1 2.6,15.34 15.56,2.38 30.28,2.38 31.88,3.98 J7.7
  Bottom 0.152: v2.6,21.1 v4.52,21.1
MOSI
  Top 0.152: IC11.34 5.64,26.06 4.2,26.06 2.6,24.46 2.6,22.06 1.96,21.42 1.96,15.5 15.4,2.06 32.52,2.06 34.44,3.98 J7.8
N$8  (via drill 2 pad 3)
  other vias: 48.28,3.05
N$9  (via drill 2 pad 3)
  other vias: 48.48,57.16
N$12  (via drill 0.35)
  Top 0.152: v23.08,19.5 24.84,19.5 CN1.7 | v31.24,19.5 32.2,19.5 R1.7
  Bottom 0.152: v31.24,19.5 v23.08,19.5
N$36  (via drill 0.35)
  Top 0.152: v12.2,38.06 11.72,38.54 11.72,39.5 C23.1 | C21.1 15.24,39.5 14.28,38.54 v14.28,38.06 12.68,36.46 12.68,33.26 14.12,31.82 v14.12,30.22 | v14.44,27.18 14.12,26.86 14.12,23.66 10.76,20.3 10.76,17.26 IC11.55
  Bottom 0.152: v14.28,38.06 v12.2,38.06 | v14.44,27.18 14.12,27.5 v14.12,30.22
N$39  (via drill 0.35)
  Top 0.152: v9.64,38.7 10.44,39.5 C26.1 | v4.52,38.7 3.56,39.66 3.56,43.02 4.04,43.5 5.48,43.5 5.96,43.02 5.96,40.94 6.6,40.3 C25.1 | v11.24,27.18 11.72,27.66 11.72,28.46 IC11.24
  Bottom 0.152: v4.52,38.7 5.8,38.7 | 5.8,38.7 v9.64,38.7 | v11.24,27.18 7.88,30.54 7.88,36.46 6.12,36.46 5.8,36.78 5.8,38.7
N$42  (via drill 0.35)
  Top 0.152: v9.16,27.18 9.8,27.82 9.8,28.46 IC11.28 | v6.92,27.34 6.92,30.22 4.84,32.3 4.84,37.42 C28.2
  Bottom 0.152: v9.16,27.18 9,27.34 v6.92,27.34
N$43  (via drill 0.35)
  Top 0.152: v11.88,36.14 12.84,37.1 12.84,39.5 C15.2 | v10.6,36.14 10.6,31.18 8.84,29.42 8.84,28.62 IC11.30
  Bottom 0.152: v10.6,36.14 v11.88,36.14
N$57  (via drill 0.35)
  Top 0.152: 8.84,39.5 8.2,39.5 R6.2 | 8.84,39.5 9.16,39.5 C30.2 | v8.84,38.06 8.84,39.5 | v16.04,17.42 16.04,17.74 15.56,18.22 15.08,18.22 14.76,17.9 14.76,17.26 | 14.76,17.26 14.28,17.26 IC11.62 | 14.76,17.26 IC11.63
  Bottom 0.152: v8.84,38.06 9.96,38.06 10.28,38.38 10.28,39.34 4.2,39.34 3.88,39.02 3.88,26.7 6.76,26.7 v16.04,17.42
N$97  (via drill 0.35)
  Top 0.152: v13.32,33.58 16.52,36.78 16.52,39.5 C14.2 | v11.4,33.58 11.4,30.06 10.76,29.42 10.76,28.62 IC11.26
  Bottom 0.152: v11.4,33.58 v13.32,33.58
NC
  Top 0.152: IC11.29 9.32,28.62 9.32,29.42 9.48,29.58 10.12,29.58 10.28,29.42 10.28,28.62 IC11.27
RESET  (via drill 0.35)
  Top 0.152: v7.08,25.26 6.92,25.1 5.8,25.1 IC11.36 | v3.4,26.22 3.4,36.78 2.6,37.58 2.6,44.46 15.88,57.74 30.12,57.74 31.72,56.14 J3.5
  Bottom 0.152: v7.08,25.26 6.12,26.22 v3.4,26.22
SCLK  (via drill 0.35)
  Top 0.152: v4.52,22.7 4.84,23.02 5.64,23.02 IC11.40 | v3.24,22.7 3.24,15.18 15.72,2.7 28.04,2.7 29.32,3.98 J7.6
  Bottom 0.152: v3.24,22.7 v4.52,22.7
SRB1  (via drill 0.35)
  Top 0.152: 34.6,36.46 34.12,36.46 R5.4 | 34.6,36.46 35.08,35.98 37.48,35.98 38.92,37.42 39.4,37.42 IC10.5 | 34.6,36.46 34.6,38.06 35.24,38.7 v35.24,39.18
  Bottom 0.152: v35.24,39.18 38.76,42.7 44.52,42.7 J2.2
SRB2  (via drill 0.35)
  Top 0.152: 39.72,35.82 40.52,36.62 40.52,37.26 40.68,37.42 41.32,37.42 IC10.2 | 39.72,35.82 39.56,35.66 34.12,35.66 R5.3 | 39.72,35.82 v39.56,35.98
  Bottom 0.152: v39.56,35.98 42.92,35.98 43.08,36.14 48.68,36.14 48.68,41.26 47.24,42.7 J2.1
(copper drawn outside any net)
  shapes: Top area x1

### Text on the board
space: AVSS | AVDD | DVDD | D18 | D13 | EN | ADS-RST | CLK | CS2 | CS1 | BIAS-INV | MCLR | 3V3 | GND | PGD | PGC | SCLK | MISO | MOSI | RXD | TXD | N/A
